| TEXAS INSTRUMENTS INCORPORATED
| Standard Linear and Logic Group
| IBIS Model of SN74CB3T3253
| 3.3-V LOW-VOLTAGE DUAL 1-OF-4 FET MULTIPLEXER/DEMULTIPLEXER
| This file contains package information for the following:
|  SOIC 16-pin (D) package as [Component] CBTLV3253_D
|  QSOP 16-pin (DBQ) package as [Component] CB3T3253_DBQ
|  TVSOP 16-pin (DGV) package as [Component] CB3T3253_DGV
|  TSSOP 16-pin (PW) package as [Component] CB3T3253_PW
| This device can be powered at the following Vccs:
|  3.3 volt Vcc
|  2.5 volt Vcc
| This file provides unique models under the [Model Selector] for each Vcc.
| For operation at a specific Vcc, select the appropriate model after each
| [Model Selector] keyword.
[IBIS Ver]   3.2
[Comment char]  |_char
[File Name]   sn74cb3t3253.ibs
[File Rev]   1.2 | a_die
[Date]   August 28, 2003
[Source]   Data created from TI-SPICE simulations at TI-SLL.
[Notes]   The following is an IBIS list for the SN74CB3T3253.
   Please contact sllibis@ti.com with questions and
   comments concerning SLL IBIS models.
   -Non-monotonic data due to FET characteristics.
   -C_comp values are taken at a different test condition than
   the Ci/Cio in data sheet.
   -Power-clamp data has been deleted since there is no
   power-clamp diode in the device.
[Disclaimer] Property of Texas Instruments Incorporated. Unauthorized
   reproduction and/or distribution is strictly prohibited.
   This product is protected under copyright law.
   Created 2002, (C) Copyright  2002, Texas Instruments
   Incorporated, All Rights Reserved
   UNLESS THERE IS A SIGNED, WRITTEN AGREEMENT TO THE
   CONTRARY, TEXAS INSTRUMENTS (TI) IS PROVIDING THE IBIS
   MODELS AND WITHOUT ANY WARRANTY, EXPRESSED OR
   IMPLIED. TI assumes no liability for:
   1) the accuracy of the IBIS models provided to your
   company;
   2) the proper functioning of these IBIS Models in your
   design or for any resulting applications; or
   3) infringement of patents, copyrights or intellectual
   property rights resulting from your use of these IBIS
   models.
   TI provides IBIS Models as a service to our customers.
   You and your company shall not distribute, sell or give
   these models to anyone else without prior written
   permission from TI.
   TI reserves the right to make changes to our products or
   to discontinue any semiconductor product or service
   without notice, and advises our customers to obtain the
   latest version of relevant information to verify, before
   placing orders, that the information being relied on is
   current.
   Please be aware that your receipt and use of the IBIS
   information provided shall serve as acceptance of these
   terms and conditions. If you do not accept these terms,
   you should return or destroy the IBIS models and any
   other accompanying information immediately.
| Component CB3T3253_D 16-pin SOIC
[Component]   CB3T3253_D
[Manufacturer]   Texas Instruments, Inc.
[Package]
|   typ   min   max
R_pkg   3.900e-02   2.800e-02   4.900e-02
L_pkg   3.453e-09   2.350e-09   4.375e-09
C_pkg   5.210e-13   2.540e-13   7.080e-13
[Pin]   signal_name   model_name   R_pin   L_pin   C_pin
1   1NOE   CB3T3253_IN   4.200e-02   4.336e-09   7.030e-13
2   S1   CB3T3253_IN   4.900e-02   3.778e-09   6.340e-13
3   1B4   CB3T3253_IO   2.800e-02   3.449e-09   5.180e-13
4   1B3   CB3T3253_IO   2.900e-02   2.393e-09   2.540e-13
5   1B2   CB3T3253_IO   2.800e-02   2.350e-09   2.640e-13
6   1B1   CB3T3253_IO   4.800e-02   3.312e-09   4.830e-13
7   1A   CB3T3253_IO   4.300e-02   3.629e-09   6.040e-13
8   GND   GND   4.400e-02   4.375e-09   7.080e-13
9   2A   CB3T3253_IO   4.200e-02   4.336e-09   7.030e-13
10   2B1   CB3T3253_IO   4.900e-02   3.778e-09   6.340e-13
11   2B2   CB3T3253_IO   2.800e-02   3.449e-09   5.180e-13
12   2B3   CB3T3253_IO   2.900e-02   2.393e-09   2.550e-13
13   2B4   CB3T3253_IO   2.800e-02   2.350e-09   2.640e-13
14   S0   CB3T3253_IN   4.800e-02   3.312e-09   4.830e-13
15   2NOE   CB3T3253_IN   4.300e-02   3.629e-09   6.040e-13
16   VCC   POWER   4.400e-02   4.375e-09   7.080e-13
| Component CB3T3253_DBQ 16-pin QSOP
[Component]   CB3T3253_DBQ
[Manufacturer]   Texas Instruments, Inc.
[Package]
|   typ   min   max
R_pkg   3.800e-02   2.700e-02   5.900e-02
L_pkg   2.353e-09   1.491e-09   4.500e-09
C_pkg   2.100e-13   6.400e-14   5.920e-13
[Pin]   signal_name   model_name   R_pin   L_pin   C_pin
1   1NOE   CB3T3253_IN   5.800e-02   4.450e-09   5.920e-13
2   S1   CB3T3253_IN   4.000e-02   1.930e-09   1.110e-13
3   1B4   CB3T3253_IO   2.800e-02   1.538e-09   7.600e-14
4   1B3   CB3T3253_IO   2.700e-02   1.491e-09   6.400e-14
5   1B2   CB3T3253_IO   2.700e-02   1.491e-09   6.400e-14
6   1B1   CB3T3253_IO   2.700e-02   1.506e-09   7.500e-14
7   1A   CB3T3253_IO   3.300e-02   1.922e-09   1.090e-13
8   GND   GND   5.900e-02   4.500e-09   5.880e-13
9   2A   CB3T3253_IO   5.800e-02   3.695e-09   4.140e-13
10   2B1   CB3T3253_IO   3.400e-02   2.685e-09   2.820e-13
11   2B2   CB3T3253_IO   2.900e-02   1.552e-09   7.700e-14
12   2B3   CB3T3253_IO   2.800e-02   1.506e-09   6.500e-14
13   2B4   CB3T3253_IO   2.700e-02   1.492e-09   6.400e-14
14   S0   CB3T3253_IN   2.800e-02   1.534e-09   7.600e-14
15   2NOE   CB3T3253_IN   4.000e-02   2.703e-09   2.840e-13
16   VCC   POWER   5.600e-02   3.645e-09   4.180e-13
| Component CB3T3253_DGV 16-pin TVSOP
[Component]   CB3T3253_DGV
[Manufacturer]   Texas Instruments, Inc.
[Package]
|   typ   min   max
R_pkg   3.900e-02   3.300e-02   4.500e-02
L_pkg   2.543e-09   2.320e-09   2.938e-09
C_pkg   3.860e-13   3.340e-13   4.490e-13
[Pin]   signal_name   model_name   R_pin   L_pin   C_pin
1   1NOE   CB3T3253_IN   3.500e-02   2.907e-09   4.170e-13
2   S1   CB3T3253_IN   4.200e-02   2.558e-09   4.460e-13
3   1B4   CB3T3253_IO   3.800e-02   2.341e-09   3.450e-13
4   1B3   CB3T3253_IO   3.800e-02   2.320e-09   3.340e-13
5   1B2   CB3T3253_IO   3.900e-02   2.322e-09   3.340e-13
6   1B1   CB3T3253_IO   3.800e-02   2.353e-09   3.420e-13
7   1A   CB3T3253_IO   4.000e-02   2.536e-09   4.410e-13
8   GND   GND   3.300e-02   2.897e-09   4.180e-13
9   2A   CB3T3253_IO   3.500e-02   2.927e-09   4.190e-13
10   2B1   CB3T3253_IO   4.500e-02   2.632e-09   4.490e-13
11   2B2   CB3T3253_IO   3.900e-02   2.368e-09   3.470e-13
12   2B3   CB3T3253_IO   3.900e-02   2.330e-09   3.350e-13
13   2B4   CB3T3253_IO   3.900e-02   2.320e-09   3.350e-13
14   S0   CB3T3253_IN   3.900e-02   2.361e-09   3.450e-13
15   2NOE   CB3T3253_IN   4.100e-02   2.573e-09   4.460e-13
16   VCC   POWER   3.500e-02   2.938e-09   4.200e-13
| Component CB3T3253_PW 16-pin TSSOP
[Component]   CB3T3253_PW
[Manufacturer]   Texas Instruments, Inc.
[Package]
|   typ   min   max
R_pkg   4.500e-02   3.800e-02   5.100e-02
L_pkg   2.593e-09   2.447e-09   3.080e-09
C_pkg   2.810e-13   2.430e-13   3.770e-13
[Pin]   signal_name   model_name   R_pin   L_pin   C_pin
1   1NOE   CB3T3253_IN   4.000e-02   3.080e-09   3.770e-13
2   S1   CB3T3253_IN   3.800e-02   2.458e-09   2.810e-13
3   1B4   CB3T3253_IO   5.100e-02   2.512e-09   2.550e-13
4   1B3   CB3T3253_IO   5.100e-02   2.447e-09   2.430e-13
5   1B2   CB3T3253_IO   5.100e-02   2.447e-09   2.430e-13
6   1B1   CB3T3253_IO   5.100e-02   2.512e-09   2.550e-13
7   1A   CB3T3253_IO   3.800e-02   2.458e-09   2.810e-13
8   GND   GND   4.000e-02   3.080e-09   3.770e-13
9   2A   CB3T3253_IO   3.900e-02   2.832e-09   3.160e-13
10   2B1   CB3T3253_IO   3.800e-02   2.460e-09   2.790e-13
11   2B2   CB3T3253_IO   5.100e-02   2.512e-09   2.550e-13
12   2B3   CB3T3253_IO   5.100e-02   2.447e-09   2.430e-13
13   2B4   CB3T3253_IO   5.100e-02   2.447e-09   2.430e-13
14   S0   CB3T3253_IN   5.100e-02   2.512e-09   2.550e-13
15   2NOE   CB3T3253_IN   3.800e-02   2.459e-09   2.790e-13
16   VCC   POWER   3.900e-02   2.832e-09   3.160e-13
[Series Switch Groups]
| Function Group States
On  1 /   | 1A->1B1 NOE1 LOW, S1 LOW, S0 LOW
On  2 /   | 1A->1B2 NOE1 LOW, S1 LOW, S0 HIGH
On  3 /   | 1A->1B3 NOE1 LOW, S1 HIGH, S0 LOW
On  4 /   | 1A->1B4 NOE1 LOW, S1 HIGH, S0 HIGH
On  5 /   | 2A->2B1 NOE2 LOW, S1 LOW, S0 LOW
On  6 /   | 2A->2B2 NOE2 LOW, S1 LOW, S0 HIGH
On  7 /   | 2A->2B3 NOE2 LOW, S1 HIGH, S0 LOW
On  8 /   | 2A->2B4 NOE2 LOW, S1 HIGH, S0 HIGH
On  1 5 /   | Enable 1 5
On  2 6 /   | Enable 2 6
On  3 7 /   | Enable 3 7
On  4 8 /   | Enable 4 8
Off 1 2 3 4 5 6 7 8 /  | Disable All
[Series Pin Mapping]   pin_2   model_name   function_table_group
7   6   CB3T3253_IO_33_S   1
| 7   6   CB3T3253_IO_25_S   1
7   5   CB3T3253_IO_33_S   2
| 7   5   CB3T3253_IO_25_S   2
7   4   CB3T3253_IO_33_S   3
| 7   4   CB3T3253_IO_25_S   3
7   3   CB3T3253_IO_33_S   4
| 7   3   CB3T3253_IO_25_S   4
9   10   CB3T3253_IO_33_S   5
| 9   10   CB3T3253_IO_25_S   5
9   11   CB3T3253_IO_33_S   6
| 9   11   CB3T3253_IO_25_S   6
9   12   CB3T3253_IO_33_S   7
| 9   12   CB3T3253_IO_25_S   7
9   13   CB3T3253_IO_33_S   8
| 9   13   CB3T3253_IO_25_S   8
| Model CB3T3253_IN
[Model Selector]   CB3T3253_IN
CB3T3253_IN_33   3.3 volt Vcc
CB3T3253_IN_25   2.5 volt Vcc
| Model CB3T3253_IO
[Model Selector]   CB3T3253_IO
CB3T3253_IO_33   3.3 volt Vcc
CB3T3253_IO_25   2.5 volt Vcc
| Model CB3T3253_IO_S
[Model Selector]   CB3T3253_IO_S
CB3T3253_IO_33_S   3.3 volt Vcc
CB3T3253_IO_25_S   2.5 volt Vcc
[Model]   CB3T3253_IO_33_S
Model_type  Series_switch
| variable   typ   min   max
C_comp   0   0   0
[Temperature Range]   40   100   -40
| Ambient temperature   25   85   -40
[Voltage range]   3.3   3   3.6
[On]
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[Off]
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[Model]   CB3T3253_IO_25_S
Model_type  Series_switch
| variable   typ   min   max
C_comp   0   0   0
[Temperature Range]   40   100   -40
| Ambient temperature   25   85   -40
[Voltage range]   2.5   2.3   2.7
[On]
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[Off]
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| Models and submodels in the file (6): CB3T3253_IN_33 (Input), CB3T3253_IN_25 (Input), CB3T3253_IO_33_S (Series_switch), CB3T3253_IO_33 (Terminator), CB3T3253_IO_25_S (Series_switch), CB3T3253_IO_25 (Terminator)
